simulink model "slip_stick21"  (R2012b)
settings: Solver=ode2  StartTime=0.0  StopTime=100  FixedStep=0.001  MaxStep=0.001  RelTol=1e-3
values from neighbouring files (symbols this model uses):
  FG = 500    [coulomb_1.m]    (also in coulomb_10.m = 10; coulomb_11.m = 10; coulomb_2.m; coulomb_3.m)
  FH = 12    [coulomb_10.m]    (also in coulomb_11.m; coulomb_3.m = 600; coulomb_4.m = 600; position_reg_1.m = 3.956)
  k = 10    [coulomb_10.m]    (also in coulomb_11.m; diff_filter_1.m = 250; diff_filter_2.m = 250; dry_friction_1.m = 2200)
  m = 400    [coulomb_1.m]    (also in coulomb_10.m = 10; coulomb_11.m = 10; coulomb_2.m; coulomb_3.m)
  sigma_0 = 5000    [position_reg_1.m]    (also in position_reg_2.m; slip_stick_21.m = 10000; slip_stick_s_12.m = 10000; tilger_gleitreib2.m = 1000)
  sigma_1 = sqrt(sigma_0)    [position_reg_1.m]    (also in position_reg_2.m; slip_stick_21.m = sqrt(1e5); slip_stick_s_12.m = sqrt(1e5); tilger_gleitreib2.m)
  sigma_2 = 0    [position_reg_1.m]    (also in position_reg_2.m; slip_stick_21.m; slip_stick_s_12.m; tilger_gleitreib2.m)
  vs = 0.05    [position_reg_1.m]    (also in position_reg_2.m; slip_stick_21.m; slip_stick_3.m = 0.01; slip_stick_31.m)
  vz = -ampl*2*pi*fanr*sin(2*pi*fanr*t)    [foerder_haft_gleit_1.m]    (also in foerder_haft_gleit_2.m; slip_stick_1.m = 0.1; slip_stick_2.m = 0.1; slip_stick_21.m = 0.1)

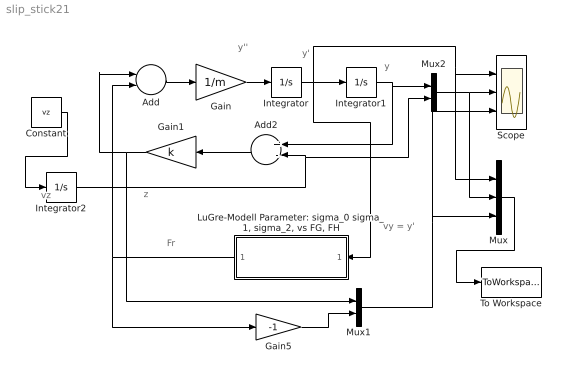
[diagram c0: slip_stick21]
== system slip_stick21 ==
  note: vy = y'
  note: z
  note: y''
  note: y'
  note: y
  note: vz
  note: Fr
  Add : Sum  Inputs=--
  Add2 : Sum  Inputs=+-
  Constant : Constant  Value=vz
  Gain : Gain  Gain=1/m
  Gain1 : Gain  Gain=k
  Gain5 : Gain  Gain=-1
  Integrator : Integrator
  Integrator1 : Integrator
  Integrator2 : Integrator
  "LuGre-Modell Parameter: sigma_0 sigma_1, sigma_2, vs FG, FH" : Subsystem
  Mux : Mux  Inputs=3
  Mux1 : Mux  Inputs=2
  Mux2 : Mux  Inputs=2
  Scope : Scope  NumInputPorts=3
  To Workspace : ToWorkspace  VariableName=y  SampleTime=-1  SaveFormat=Structure With Time
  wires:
  Add/1 -> Gain/1
  Gain/1 -> Integrator/1
  "LuGre-Modell Parameter: sigma_0 sigma_1, sigma_2, vs FG, FH"/1(Fr) -> Add/2, Gain5/1
  Gain1/1 -> Add/1, Mux1/1
  Mux1/1 -> Scope/3, Mux/3
  Gain5/1 -> Mux1/2
  Mux/1 -> To Workspace/1
  Constant/1 -> Integrator2/1
  Integrator1/1 -> Add2/1, Mux2/1
  Integrator/1 -> "LuGre-Modell Parameter: sigma_0 sigma_1, sigma_2, vs FG, FH"/1(v), Integrator1/1, Mux/1, Scope/1
  Mux2/1 -> Mux/2, Scope/2
  Add2/1 -> Gain1/1
  Integrator2/1 -> Mux2/2, Add2/2

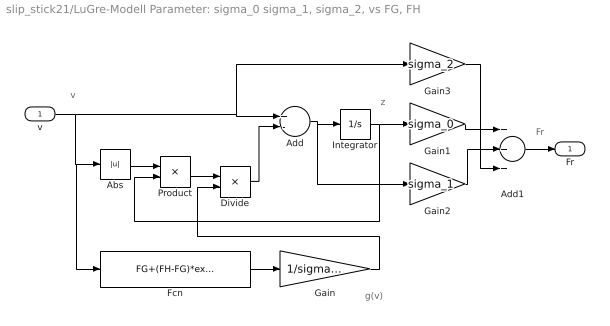
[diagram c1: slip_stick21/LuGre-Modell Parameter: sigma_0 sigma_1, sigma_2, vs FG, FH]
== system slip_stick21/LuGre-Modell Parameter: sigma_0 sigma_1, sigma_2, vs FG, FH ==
  note: z
  note: g(v)
  note: v
  note: Fr
  v : Inport
  Abs : Abs
  Add : Sum  Inputs=+-
  Add1 : Sum  Inputs=+++
  Divide : Product  Inputs=*/
  Fcn : Fcn  Expr=FG+(FH-FG)*exp(-(u/vs)^2)
  Gain : Gain  Gain=1/sigma_0
  Gain1 : Gain  Gain=sigma_0
  Gain2 : Gain  Gain=sigma_1
  Gain3 : Gain  Gain=sigma_2
  Integrator : Integrator
  Product : Product
  Fr : Outport
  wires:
  Product/1 -> Divide/1
  Gain/1 -> Divide/2
  Fcn/1 -> Gain/1
  Gain3/1 -> Add1/3
  Add1/1 -> Fr/1
  Gain1/1 -> Add1/1
  Divide/1 -> Add/2
  Abs/1 -> Product/1
  Gain2/1 -> Add1/2
  Add/1 -> Integrator/1, Gain2/1
  Integrator/1 -> Product/2, Gain1/1
  v/1 -> Abs/1, Fcn/1, Add/1, Gain3/1
